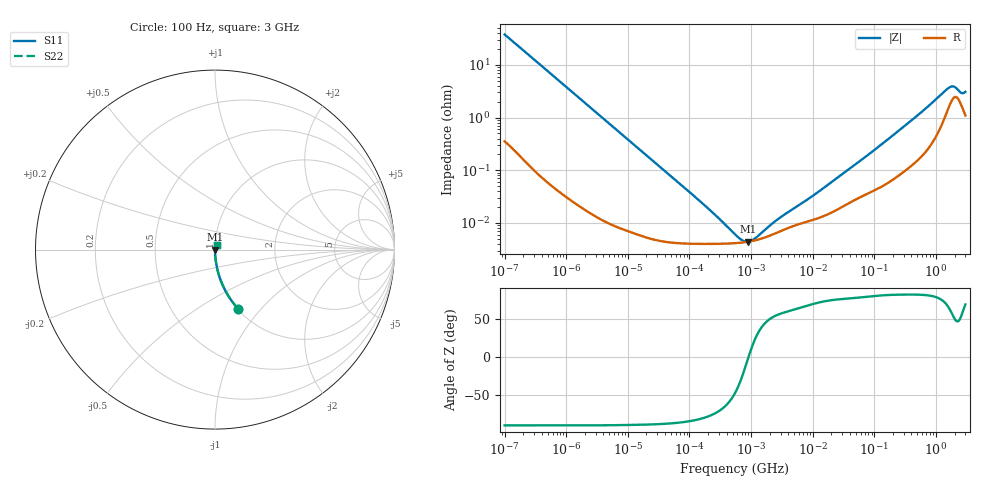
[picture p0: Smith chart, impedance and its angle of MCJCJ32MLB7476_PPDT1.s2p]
! MCJCJ32MLB7476_PPDT1  S-PARAMETER MODEL  ( Standard Model )
! Model Generated by TAIYO YUDEN Corporation (http://www.ty-top.com)
! Version 2.0
! TAIYO YUDEN Control No. 240725
! Copyright(c) 2015 TAIYO YUDEN CO.,LTD. All Rights Reserved.
! Product Description (link to TY-COMPAS)
! https://ds.yuden.co.jp/TYCOMPAS/or/detail?pn=MCJCJ32MLB7476KPPDT1&u=M
! Products Name : Multilayer Ceramic Capacitors
! Characteristics :
!  Capacitance : 47 [uF] , Rated Voltage : 6.3 [V] , TCC : X7R
!  Case Size : 3.2 x 2.5 / 0.126 x 0.098 [mm/inch] , Thickness : 2.5 / 0.098 [mm/inch]
!  (Conditions: Temperature = 25 [degC] , DC Bias Voltage = 0 [V])
! External Node Assignments :
!  1  o---| |---o  2
! GND o---------o GND
! Frequency Range : 100Hz  -  3GHz  [ 401 STEP ]
# MHZ S RI R 50
! Freq[MHz].  S11 Real  S11 Imag  S21 Real  S21 Imag  S12 Real  S12 Imag  S22 Real  S22 Imag
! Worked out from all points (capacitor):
!   401 points, 100 Hz to 3 GHz, reference 50 ohm
!   read as one part in series: C = 42 uF near 109 Hz
!   lowest |Z| = 4.41 mohm at 879.4 kHz (marker M1)
!   series resonance near 906 kHz, so ESL is about 730 pH
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0.0001  0.1275 -0.3288  0.8725 0.3288  0.8725 0.3288  0.1275 -0.3288
0.000175  0.0466 -0.2065  0.9534 0.2065  0.9534 0.2065  0.0466 -0.2065
0.000348  0.0126 -0.1079  0.9874 0.1079  0.9874 0.1079  0.0126 -0.1079
0.000724  0.00318 -0.0526  0.9968 0.0526  0.9968 0.0526  0.00318 -0.0526
0.001788  0.000653 -0.0214  0.9993 0.0214  0.9993 0.0214  0.000653 -0.0214
0.031977  4.76e-05 -0.00122  1 0.00122  1 0.00122  4.76e-05 -0.00122
0.138163  4.03e-05 -0.000276  1 0.000276  1 0.000276  4.03e-05 -0.000276
0.341146  4.04e-05 -9.78e-05  1 9.78e-05  1 9.78e-05  4.04e-05 -9.78e-05
0.388167  4.06e-05 -8.16e-05  1 8.16e-05  1 8.16e-05  4.06e-05 -8.16e-05
0.547723  4.14e-05 -4.47e-05  1 4.47e-05  1 4.47e-05  4.14e-05 -4.47e-05
0.87939  4.4e-05 -2.49e-06  1 2.49e-06  1 2.49e-06  4.4e-05 -2.49e-06
2.266852  6.09e-05 7.98e-05  0.9999 -7.98e-05  0.9999 -7.98e-05  6.09e-05 7.98e-05
9.794414  0.000113 0.000301  0.9999 -0.000301  0.9999 -0.000301  0.000113 0.000301
67.94454  0.000337 0.00168  0.9997 -0.00168  0.9997 -0.00168  0.000337 0.00168
175.1444  0.000615 0.00403  0.9994 -0.00403  0.9994 -0.00403  0.000615 0.00403
536.3016  0.00179 0.0116  0.9982 -0.0116  0.9982 -0.0116  0.00179 0.0116
1382.454  0.0107 0.0296  0.9893 -0.0296  0.9893 -0.0296  0.0107 0.0296
1642.185  0.0173 0.0324  0.9827 -0.0324  0.9827 -0.0324  0.0173 0.0324
1789.813  0.0212 0.0318  0.9788 -0.0318  0.9788 -0.0318  0.0212 0.0318
1950.712  0.0242 0.0292  0.9758 -0.0292  0.9758 -0.0292  0.0242 0.0292
2525.516  0.0184 0.0227  0.9816 -0.0227  0.9816 -0.0227  0.0184 0.0227
3000  0.0117 0.0282  0.9883 -0.0282  0.9883 -0.0282  0.0117 0.0282
